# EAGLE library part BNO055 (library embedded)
BREAKOUT BOARD Adafruit BNO055 Absolute Orientation Sensor https://learn.adafruit.com/adafruit-bno055-absolute-orientation-sensor/overview
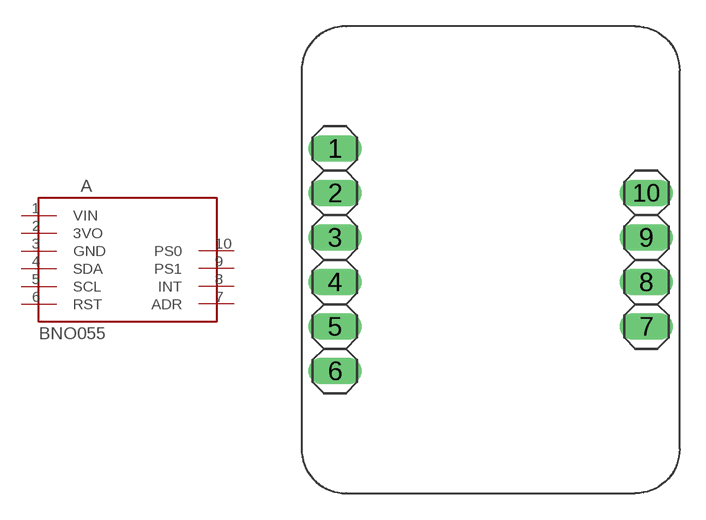
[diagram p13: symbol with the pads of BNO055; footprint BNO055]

Designator prefix A

## BNO055 (DATASHEET: https://cdn-learn.adafruit.com/downloads/pdf/adafruit-bno055-absolute-orientation-sensor.pdf; DESCR: Acceleration Sensor Development Tools Adafruit 9-DOF Absolute Orientation IMU Fusion Breakout - BNO055; MF: Adafruit; MF_PN: 2472; MOUSER_NO: 485-2472; PURCHASE: https://www.reichelt.de/development-boards-sensor-with-different-functions-debo-sens-combi-p235479.html?PROVID=2788&gclid=EAIaIQobChMIppaP2Nqd4gIVA853Ch3mIQILEAYYASABEgKn7_D_BwE&&r=1; REICHELT_NO: DEBO SENS COMBI; UNIT_PRICE: 30.52)  [BNO055]
1  VIN
2  3VO
3  GND
4  SDA
5  SCL
6  RST
7  ADR
8  INT
9  PS1
10  PS0

## Footprint BNO055 (pad centres in mm)
drill 1.016 long: 1 -8.89,6.35; 2 -8.89,3.81; 3 -8.89,1.27; 4 -8.89,-1.27; 5 -8.89,-3.81; 6 -8.89,-6.35; 7 8.89,-3.81; 8 8.89,-1.27; 9 8.89,1.27; 10 8.89,3.81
